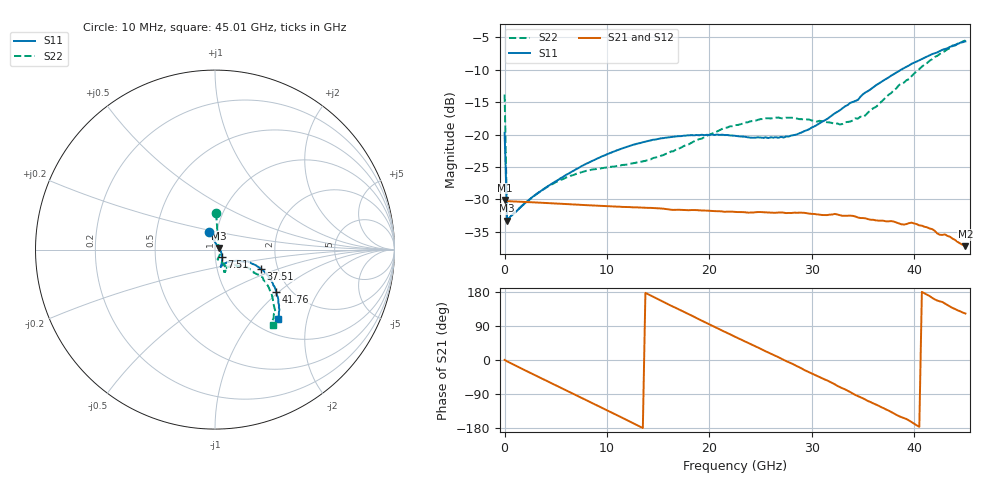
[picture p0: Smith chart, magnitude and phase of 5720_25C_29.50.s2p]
! Device:  ADRF5720
! Description: 0.5dB LSB GaAs MMIC 6-bit Digital Attenuator
! Frequency:  0.000009 -  40 GHz
! Ports:
!	RF1	= Port 1
!	RF2	= Port 2
! Vdd:  3.3 Volt
! Vss:  -3.3 Volt
! Control:  0/3.3 Volt
! State:  29.50 dB attenuation
! Data:  The device was measured using G-S-G Probes on a matrix board.
!  Data was collected using an calibrated 4 port network analyzer.
!  The reference plane for this measurement is at the launchers.
! Note:  Analog Devices supplies this data as a sample of measured data
!  for this product.  Your particular data for this product may vary.
!  Data was taken at 25 degrees C.
!  Analog Devices reserves the right to change this data at anytime.
# GHZ S DB R 45.0
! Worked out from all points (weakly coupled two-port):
!   181 points, 10 MHz to 45.01 GHz, reference 45 ohm
!   highest |S21| = -30.07 dB at 10 MHz (marker M1); lowest = -37.2 dB at 45.01 GHz (marker M2)
!   lowest |S11| = -33.2 dB at 260 MHz (marker M3), VSWR 1.04, Z = 46.8 + j0.873 ohm
!   |S11| at or under -10 dB: start of sweep to 38.74 GHz
!   |S22| runs from -33.4 to -5.5 dB; largest |S21 - S12| = 0.00011
!   S11 on the Smith chart (normalised r, x): 10 MHz: 0.92, +0.18; 7.51 GHz: 1.08, -0.09; 37.51 GHz: 1.63, -0.37; 41.76 GHz: 1.69, -0.97; 45.01 GHz: 1.27, -1.35
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0.01  -19.73 109.2  -30.07 0.2  -30.06 0.2  -13.84 88.2
0.26  -33.25 25.4  -30.26 -3.7  -30.26 -3.7  -33.44 22.5
3.26  -29.01 -18.9  -30.48 -43.9  -30.48 -43.8  -29.01 -38.8
5.01  -27.19 -32.9  -30.63 -66.9  -30.62 -66.9  -27.33 -56.4
7.51  -24.88 -46.2  -30.84 -99.7  -30.83 -99.7  -25.82 -70.0
7.76  -24.68 -47.3  -30.86 -103.0  -30.85 -103.1  -25.69 -71.0
11.51  -22.13 -59.8  -31.15 -152.6  -31.15 -152.6  -24.69 -74.2
15.26  -20.59 -67.7  -31.39 156.6  -31.39 156.7  -23.28 -65.7
20.26  -19.98 -71.3  -31.78 90.4  -31.78 90.5  -19.86 -58.8
22.76  -20.26 -69.2  -31.94 58.2  -31.94 58.2  -18.53 -60.7
25.51  -20.42 -59.6  -31.99 22.9  -31.99 23.0  -17.50 -65.0
27.26  -20.47 -51.6  -32.04 0.2  -32.06 0.2  -17.53 -66.3
30.26  -18.75 -33.6  -32.24 -38.6  -32.25 -38.6  -17.85 -65.7
32.76  -16.25 -24.2  -32.43 -71.7  -32.43 -71.6  -18.45 -56.1
33.76  -15.13 -22.6  -32.50 -84.6  -32.49 -84.6  -18.00 -47.8
35.01  -13.79 -20.2  -32.87 -101.2  -32.87 -101.1  -17.30 -40.3
37.51  -11.20 -22.7  -33.38 -133.5  -33.39 -133.4  -13.87 -29.2
37.76  -10.92 -23.2  -33.33 -137.0  -33.33 -136.9  -13.61 -28.9
40.26  -8.74 -29.7  -33.80 -172.6  -33.78 -172.8  -10.24 -30.3
41.76  -7.61 -34.8  -34.57 164.1  -34.55 164.3  -8.39 -36.6
43.76  -6.37 -42.1  -36.04 137.3  -36.05 137.3  -6.26 -46.0
45.01  -5.65 -47.9  -37.20 122.7  -37.23 122.7  -5.50 -52.6
